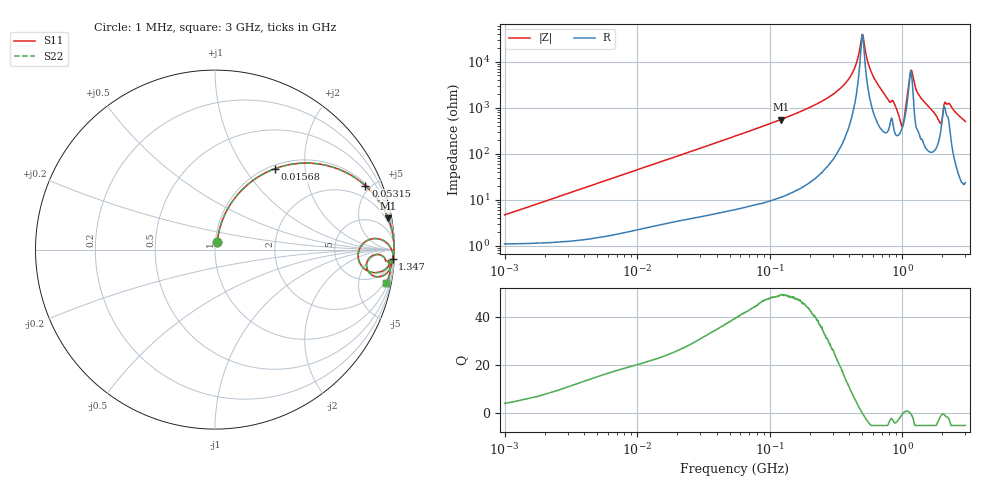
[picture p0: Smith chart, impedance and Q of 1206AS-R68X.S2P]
!s-Parameter Generated by FASTRON Sdn. Bhd.
!FASTRON P/N : 1206AS-R68X
!Keysight Technologies: E4991B_MY54100416_A.01.15
!Date created: Thu Nov 16 13:23:34 2023
!Version  : Rev00 Thu Nov 16 13:23:34 2023
!Data & Calibration Information:
!Freq	S11	S21	S12	S22
!PortZ  Port1:50+j0  Port2:50+j0
!When reading reference impedance value at option line is always used.
! Remarks : This data is being provided solely for informational purposes.
# Hz S dB R 50
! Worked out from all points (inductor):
!   1601 points, 1 MHz to 3 GHz, reference 50 ohm
!   read as one part in series: L = 728 nH near 1.041 MHz
!   highest Q = 49 at 121.4 MHz (marker M1), where L = 725 nH
!   self-resonance near 500.2 MHz
!   S11 on the Smith chart (normalised r, x): 1 MHz: 1.02, +0.09; 15.68 MHz: 1.06, +1.39; 53.15 MHz: 1.12, +4.66; 1.347 GHz: 6, -36; 3 GHz: 1, -10
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1000000  -26.65 73.9  -0.10 -2.6  -0.10 -2.6  -26.65 73.9
3804036  -15.46 75.9  -0.24 -9.7  -0.24 -9.7  -15.46 75.9
1.447069e7  -5.50 55.5  -1.67 -32.0  -1.67 -32.0  -5.50 55.5
1.567691e7  -5.03 53.5  -1.88 -34.0  -1.88 -34.0  -5.03 53.5
5.315222e7  -0.81 23.0  -8.17 -65.6  -8.17 -65.6  -0.81 23.0
5.477226e7  -0.77 22.4  -8.39 -66.2  -8.39 -66.2  -0.77 22.4
1.213667e8  -0.17 10.2  -15.02 -78.6  -15.02 -78.6  -0.17 10.2
2.083556e8  -0.06 5.3  -20.62 -83.3  -20.62 -83.3  -0.06 5.3
3.855751e8  -0.02 1.5  -31.67 -83.9  -31.67 -83.9  -0.02 1.5
4.435663e8  -0.02 0.7  -38.05 -78.9  -38.05 -78.9  -0.02 0.7
5.001674e8  -0.02 0.0  -51.82 -7.3  -51.82 -7.3  -0.02 0.0
5.929311e8  -0.03 -1.0  -34.68 78.6  -34.68 78.6  -0.03 -1.0
7.925923e8  -0.17 -3.9  -23.14 72.0  -23.14 72.0  -0.17 -3.9
8.629671e8  -0.20 -4.1  -22.58 70.0  -22.58 70.0  -0.20 -4.1
1.002744e9  -1.94 -3.4  -13.67 13.3  -13.67 13.3  -1.94 -3.4
1.048936e9  -0.90 3.9  -18.55 -31.4  -18.55 -31.4  -0.90 3.9
1.136371e9  -0.18 0.5  -32.93 -23.0  -32.93 -23.0  -0.18 0.5
1.176881e9  -0.11 -0.5  -36.26 31.2  -36.26 31.2  -0.11 -0.5
1.347129e9  -0.08 -3.1  -25.35 78.6  -25.35 78.6  -0.08 -3.1
1.902655e9  -0.79 -9.5  -14.85 56.6  -14.85 56.6  -0.79 -9.5
2.167021e9  -0.42 -3.8  -21.94 51.8  -21.94 51.8  -0.42 -3.8
3e9  -0.25 -11.1  -14.27 76.2  -14.27 76.2  -0.25 -11.1
